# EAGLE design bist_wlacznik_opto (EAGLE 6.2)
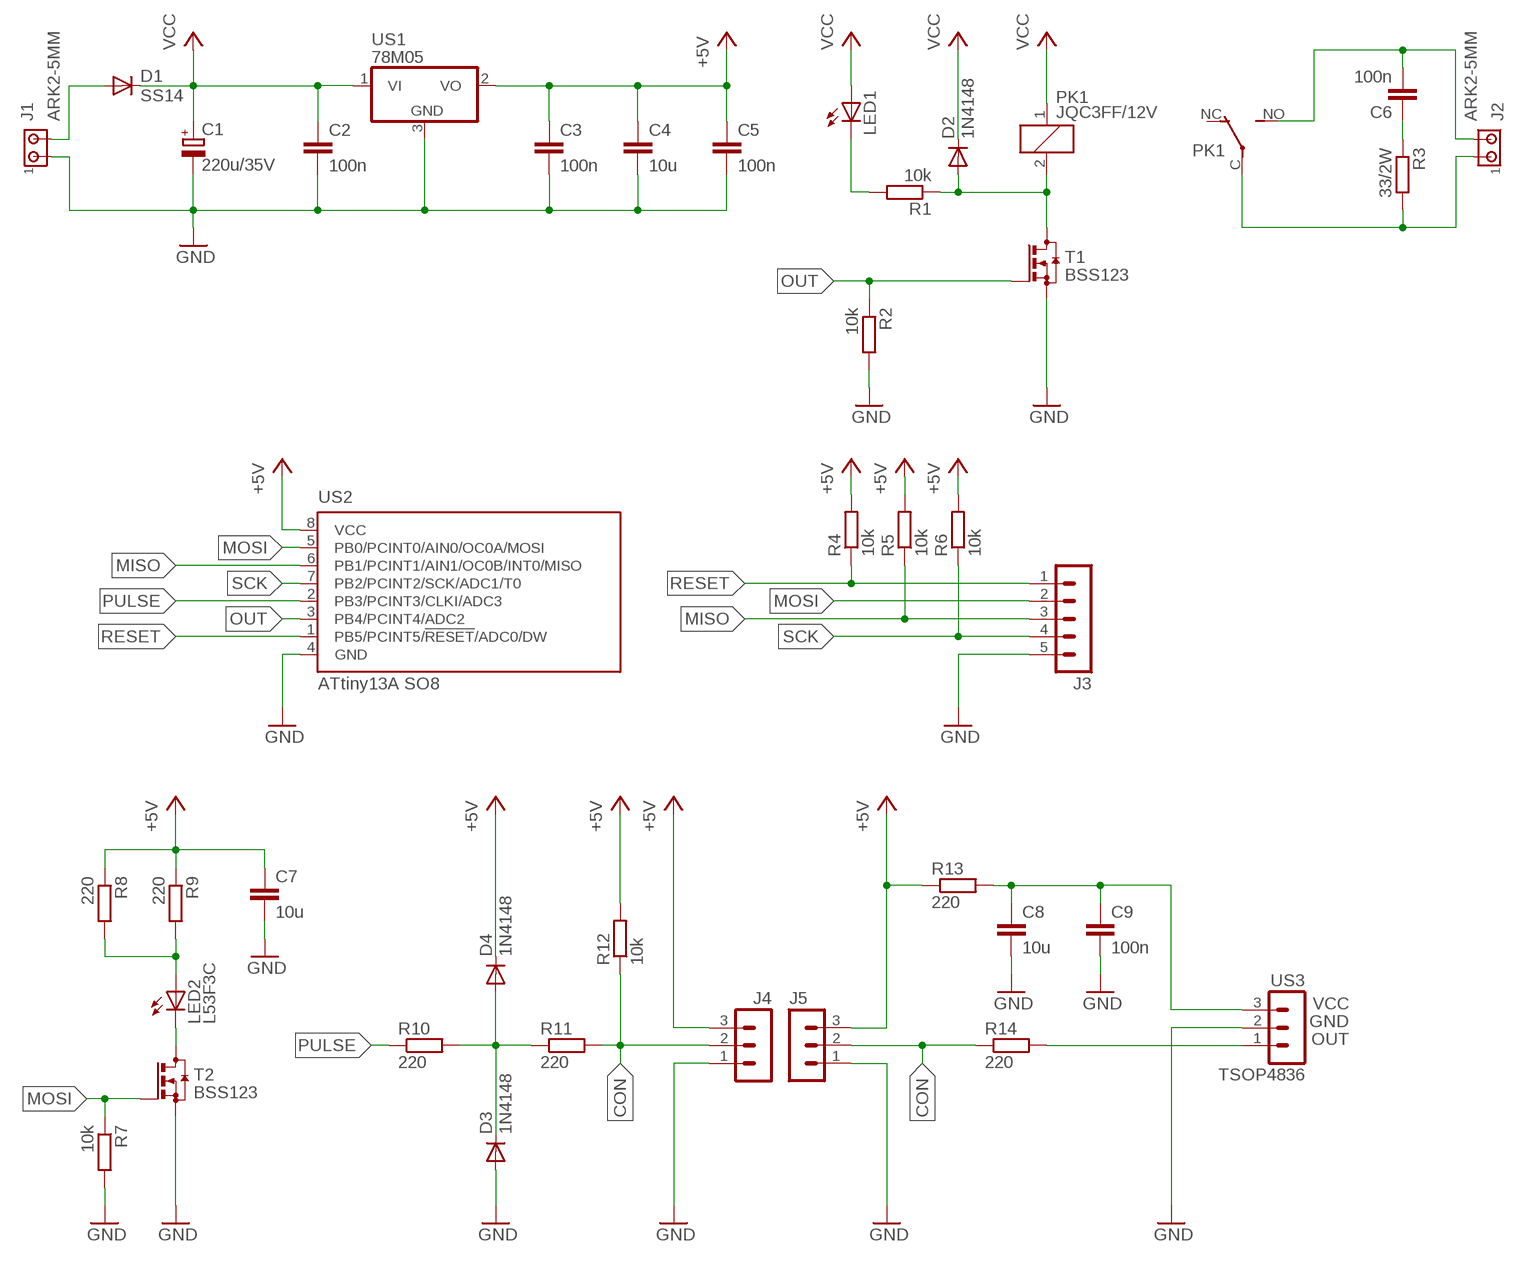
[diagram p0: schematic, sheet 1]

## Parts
C1  220u/35V  CPOL-EUE3.5-8  [E3,5-8]
C2  100n  C-EUC0805  [C0805]
C3  100n  C-EUC0805  [C0805]
C4  10u  C-EUC0805  [C0805]
C5  100n  C-EUC0805  [C0805]
C6  100n  C-EU102_152-062X184  [C102_152-062X184]
C7  10u  C-EUC0805  [C0805]
C8  10u  C-EUC0805  [C0805]
C9  100n  C-EUC0805  [C0805]
D1  SS14  DIODE-DO214AC  [DO214AC]
D2  1N4148  DIODE-MINIMELF  [MINIMELF]
D3  1N4148  DIODE-MINIMELF  [MINIMELF]
D4  1N4148  DIODE-MINIMELF  [MINIMELF]
J1  ARK2-5MM  [2PIN-5MM]
J2  ARK2-5MM  [2PIN-5MM]
J3  MA05-1  [MA05-1]
J4  MA03-1  [MA03-1]
J5  MA03-1  [MA03-1]
LED1  LEDCHIP-LED0805  [CHIP-LED0805]
LED2  L53F3C  LED5MM  [LED5MM]
PK1  JQC3FF/12V  PK_POJED-JQC-3FG  [PK_POJED_JQC-3FG]
R1  10k  R-EU_R0805  [R0805]
R2  10k  R-EU_M0805  [M0805]
R3  33/2W  R-EU_0617/5V  [0617V]
R4  10k  R-EU_R0805  [R0805]
R5  10k  R-EU_R0805  [R0805]
R6  10k  R-EU_R0805  [R0805]
R7  10k  R-EU_M0805  [M0805]
R8  220  R-EU_M0805  [M0805]
R9  220  R-EU_M0805  [M0805]
R10  220  R-EU_M0805  [M0805]
R11  220  R-EU_M0805  [M0805]
R12  10k  R-EU_R0805  [R0805]
R13  220  R-EU_M0805  [M0805]
R14  220  R-EU_M0805  [M0805]
T1  BSS123  [SOT23]
T2  BSS123  [SOT23]
US1  78M05  7806DT  [TO252]
US2  ATtiny13A SO8  TINY13V-10SSU  [8S1]
US3  TSOP4836  MA03-1  [MA03-1]

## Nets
+5V: C3.1 C4.1 C5.1 C7.1 D4.C J4.3 J5.3 R4.2 R5.2 R6.2 R8.1 R9.1 R12.2 R13.1 US1.2(VO) US2.8(VCC)
CON: J4.2 J5.2 R11.2 R12.1 R14.1
GND: C1.- C2.2 C3.2 C4.2 C5.2 C7.2 C8.2 C9.2 D3.A J1.P$1 J3.5 J4.1 J5.1 R2.2 R7.2 T1.2(S) T2.2(S) US1.3(GND) US2.4(GND) US3.2
MISO: J3.3 R5.1 US2.6(PB1/PCINT1/AIN1/OC0B/INT0/MISO)
MOSI: J3.2 R7.1 T2.1(G) US2.5(PB0/PCINT0/AIN0/OC0A/MOSI)
N$1: D1.A J1.P$2
N$2: LED1.C R1.2
N$4: LED2.K(C) T2.3(D)
N$5: LED2.A R8.2 R9.2
N$6: C8.1 C9.1 R13.2 US3.3
N$7: R14.2 US3.1
N$8: D3.C D4.A R10.2 R11.1
N$9: C6.1 R3.1
N$10: J2.P$1 PK1.C(COM) R3.2
N$11: C6.2 J2.P$2 PK1.NO
N$12: D2.A PK1.2 R1.1 T1.3(D)
OUT: R2.1 T1.1(G) US2.3(PB4/PCINT4/ADC2)
PULSE: R10.1 US2.2(PB3/PCINT3/CLKI/ADC3)
RESET: J3.1 R4.1 US2.1(PB5/PCINT5/!RESET!/ADC0/DW)
SCK: J3.4 R6.1 US2.7(PB2/PCINT2/SCK/ADC1/T0)
VCC: C1.+ C2.1 D1.C D2.C LED1.A PK1.1 US1.1(VI)
Unconnected: PK1.NC

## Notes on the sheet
- VCC
- GND
- OUT

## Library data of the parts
C1 = rcl:CPOL-EU: POLARIZED CAPACITOR, European symbol
C2-C5 C7-C9 = rcl:C-EU: CAPACITOR, European symbol
C6 = resistor:C-EU: CAPACITOR, European symbol
D1-D4 = diode:DIODE-: DIODE
J1 J2 = zlacza_futrzak:ARK2: ARK 2
J3 = zlacza_futrzak:MA05-1: PIN HEADER; OC_FARNELL: unknown; OC_NEWARK: unknown
J4 J5 = con-lstb:MA03-1: PIN HEADER; OC_FARNELL: unknown; OC_NEWARK: unknown
LED1 LED2 = led:LED: LED
PK1 = inne_futrzak:PK_POJED
R1 R2 R4-R14 = rcl:R-EU_: RESISTOR, European symbol
R3 = resistor:R-EU_: RESISTOR, European symbol
T1 T2 = transistor-small-signal:BSS123: N-CHANNEL MOS FET
US1 = linear:78*: Positive VOLTAGE REGULATOR Source: http://cache.national.com/ds/LM/LM78L05.pdf http://www.fairchildsemi.com/ds/LM/LM7805.pdf
US2 = atmel:TINY13: 8-bit AVR Microcontroller with 1K Bytes In-System Programmable Flash Source: http://www.atmel.com/dyn/resources/prod_documents/2535S.pdf; MPN: ATTINY13V-10SSU; OC_FARNELL: 1455135; OC_NEWARK: 58M3773
US3 = zlacza_futrzak:MA03-1: PIN HEADER; OC_FARNELL: unknown; OC_NEWARK: unknown

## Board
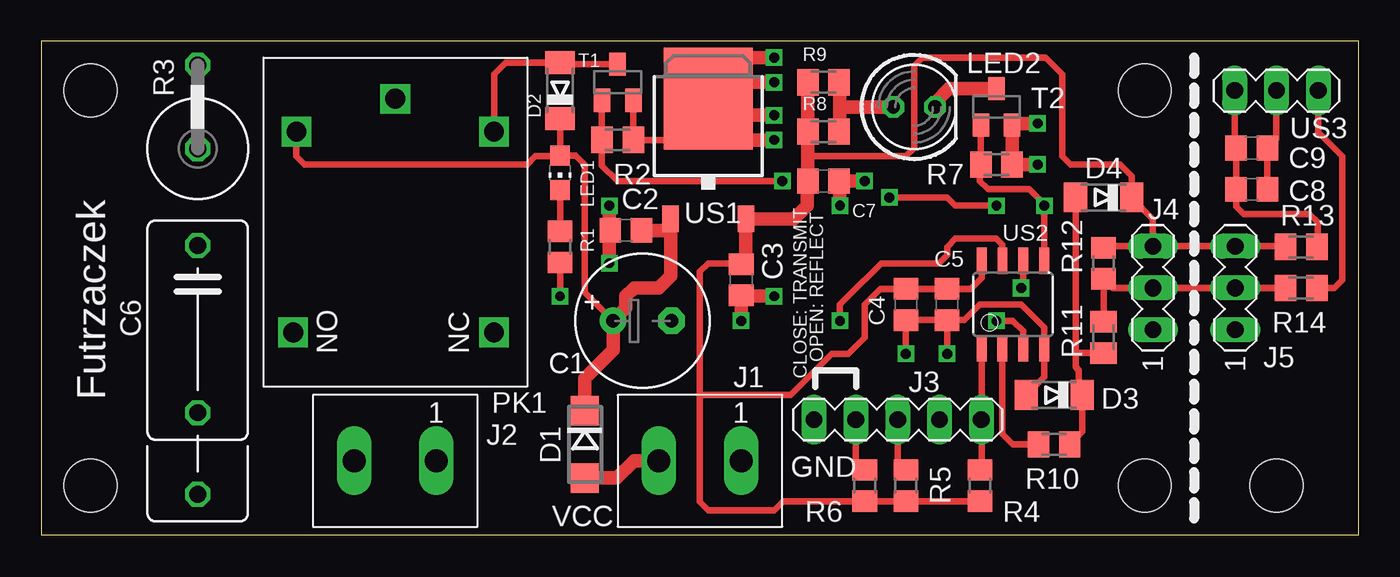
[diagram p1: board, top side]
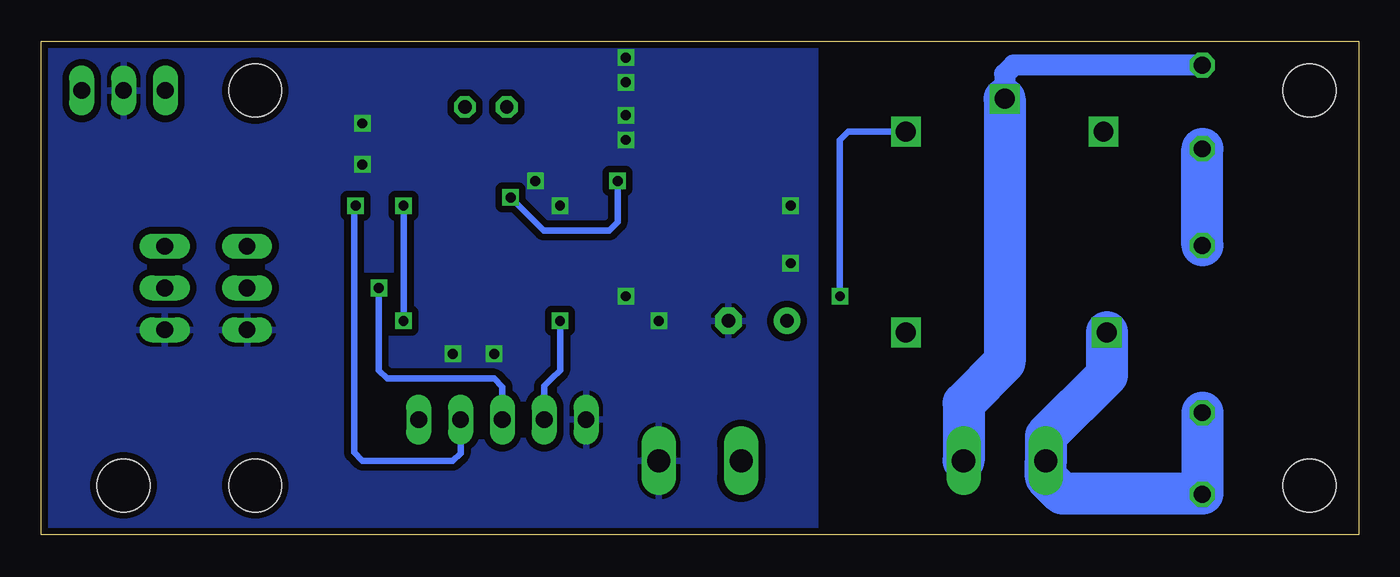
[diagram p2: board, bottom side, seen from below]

Size 80 x 30 mm. Coordinates in mm from the lower left corner, seen from the top.
Outline: 0,0 80,0 80,30 0,30 0,0
Copper layers (1*16): Top 0.035mm / dielectric 1.5mm / Bottom 0.035mm
Design rules: minimum track width 10mil, minimum drill 23mil, track to track 8mil, track to pad 8mil, pad to pad 8mil, via to via 8mil, smd to smd 8mil, copper to edge 10mil, drill to drill 8mil, minimum pad ring 10mil, minimum via ring 8mil, stop-mask expansion 4mil, vias tented up to drill 0mil, thermal gap 10mil
Holes 3.2 mm at 3,3 3,27 75,3 67,27 67,3

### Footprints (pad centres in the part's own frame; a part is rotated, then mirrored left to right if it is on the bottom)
E3,5-8 = drill 0.813 pad 1.6: + -1.778,0 | drill 0.813 pad 1.6 octagon: - 1.778,0
C0805 = smd 1.3 x 1.5: 1 -0.95,0; 2 0.95,0
C102_152-062X184 = drill 1.016 octagon: 1 -5.08,0; 2 5.08,0; 3 10.033,0
DO214AC = smd 1.8 x 1.7: A 2.05,0; C -2.05,0
MINIMELF = smd 1.4 x 1.8: A 1.7,0; C -1.7,0
2PIN-5MM = drill 1.4 long: P$1 -2.5,0; P$2 2.5,0
MA05-1 = drill 1.016 long: 1 -5.08,0; 2 -2.54,0; 3 0,0; 4 2.54,0; 5 5.08,0
MA03-1 = drill 1.016 long: 1 -2.54,0; 2 0,0; 3 2.54,0
CHIP-LED0805 = smd 1.2 x 1.2: A 0,-1.05; C 0,1.05
LED5MM = drill 0.813 octagon: A -1.27,0; K 1.27,0
PK_POJED_JQC-3FG = drill 1.2 square: 1 5.5,6; 2 5.5,-6; C 7.5,0; NC -6.7,-6; NO -6.7,6.2
R0805 = smd 1.3 x 1.5: 1 -0.95,0; 2 0.95,0
M0805 = smd 1.3 x 1.6: 1 -0.95,0; 2 0.95,0
0617V = drill 1.016 octagon: 1 -2.54,0; 2 2.54,0
SOT23 = smd 1 x 1.4: 1 -0.95,-1.1; 2 0.95,-1.1; 3 0,1.1
TO252 = smd 1 x 1.6: 1 -2.28,-4.8; 2 2.28,-4.8 | smd 5.4 x 6.2: 3 0,2.5
8S1 = smd 0.6 x 1.6: 1 -1.905,-2.654; 2 -0.645,-2.654; 3 0.625,-2.654; 4 1.895,-2.654; 5 1.905,2.654; 6 0.635,2.654; 7 -0.635,2.654; 8 -1.905,2.654

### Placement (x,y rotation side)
C1  36.5,13 0 top
C2  35.5,18.5 180 top
C3  42.5,15.5 270 top
C4  52.5,14 270 top
C5  55,14 270 top
C6  9.5,12.5 270 top
C7  47.5,21.5 0 top
C8  73.5,21 0 top
C9  73.5,23.5 0 top
D1  33,5.5 270 top
D2  31.5,27 90 top
D3  61.5,8.5 180 top
D4  64.5,20.5 180 top
J1  40,4.5 180 top
J2  21.5,4.5 180 top
J3  52,7 180 top
J4  67.5,15 90 top
J5  72.5,15 90 top
LED1  31.5,22 180 top
LED2  53,26 0 top
PK1  21.5,19 90 top
R1  31.5,17.5 90 top
R2  35,24 0 top
R3  9.5,26 90 top
R4  57,3 270 top
R5  52.5,3 270 top
R6  50,3 270 top
R7  58,22.5 0 top
R8  47.5,24.5 0 top
R9  47.5,27.5 0 top
R10  61.5,5.5 0 top
R11  64.5,12 90 top
R12  64.5,16.5 90 top
R13  76.5,17.5 0 top
R14  76.5,15 0 top
T1  35,27.5 0 top
T2  58,26 0 top
US1  40.5,24 0 top
US2  59,14 0 top
US3  75,27 180 top

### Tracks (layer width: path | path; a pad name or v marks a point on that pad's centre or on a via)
+5V
  Top 0.406: R13.1 75.51,17.54 J5.3 J4.3 | 40,8.5 40,2 40.5,1.5 44.5,1.5 45.05,2.05 R6.2 R5.2 R4.2 | 40,8.5 40,16 40.5,16.5 41.95,16.5 C3.1 | 40,8.5 45.5,8.5 47.96,10.96 48,11 49,11 50,12 50,14 50.95,14.95 C4.1 C5.1 56.45,14.95 57.09,15.6 US2.8 | J4.3 64.59,17.54 R12.2 | 46.55,23 52.5,23 53,23.5 53,28.5 53.5,29 61,29 62,28 62,23 62.5,22.5 65.5,22.5 66.2,21.8 D4.C 67.5,19.2 J4.3
  Top 0.813: R9.1 R8.1 46.55,23 C7.1 46.5,21.45 46.5,20 45.7,19.2 US1.2 42.78,16.73 C3.1
CON
  Top 0.406: R14.1 J5.2 J4.2 65.05,15 R12.1 R11.2
GND  (via drill 0.6)
  Top 0.406: T1.2 R2.2 40.5,24 | US3.2 75,24.05 C9.2 C8.2 | v52.5,11 C4.2 C5.2 | v55,11 C5.2 | D3.A 60.9,9.6 US2.4 60.9,12.61 59.5,14 57,14 56.05,13.05 C5.2
  Top 0.813: v44.5,24 40.5,24 40.5,25.5 | 40.5,25.5 US1.3 40.5,27.5 | v44.5,25.5 40.5,25.5 | v44.5,27.5 40.5,27.5 | v44.5,29 41,29 40.5,28.5 40.5,27.5 | v34.5,20 34.5,18.55 C2.2 34.5,18.45 v34.5,16.5 | 42.45,14.5 C3.2 | v42.5,13 C3.2 | v48.5,20 48.5,21.45 C7.2 v50,21.5 | v60.5,25 59.05,25 T2.2 R7.2 v60.5,22.5 | v44.5,14.5 42.55,14.5 C3.2
  pour Bottom (isolate 0.406): 80,0 80,30 33,30 33,0
MISO  (via drill 0.6)
  Top 0.406: US2.6 59.63,15.13 v59.5,15 | J3.3 52,4.45 R5.1
  Bottom 0.406: J3.3 52,9 52.5,9.5 59,9.5 59.5,10 v59.5,15
MOSI  (via drill 0.6)
  Top 0.406: T2.1 R7.1 57,22.45 57,21.5 57.5,21 60,21 60.91,20.09 v60.91,20 US2.5
  Bottom 0.406: J3.2 54.54,4.96 55,4.5 60.5,4.5 61,5 61,19.91 v60.91,20
N$1
  Top 0.813: D1.A 34.95,3.45 36,4.5 J1.P$2
N$2
  Top 0.406: R1.2 LED1.C
N$4
  Top 0.813: T2.3 55.1,27.1 54.27,26.27 LED2.K
N$5
  Top 0.813: LED2.A 48.5,26 | 48.5,26 48.5,24.55 R8.2 | 48.5,26 48.5,27.45 R9.2
N$6
  Top 0.406: US3.3 72.46,23.59 C9.1 C8.1 72.55,19.95 73,19.5 77,19.5 77.5,19 77.5,17.55 R13.2
N$7
  Top 0.406: R14.2 78.5,15 79,15.5 79,23 77.54,24.46 US3.1
N$8
  Top 0.406: R10.2 63.2,6.25 D3.C 63,8.7 63,10 62.8,10.2 62.8,11 | D4.A 62.8,11 | R11.1 62.85,11.05 62.8,11
N$9
  Bottom 2.54: C6.1 R3.1
N$10
  Bottom 1.27: R3.2 20.96,28.54 21.5,28 PK1.C
  Bottom 2.54: PK1.C 21.5,10.5 24,8 J2.P$1
N$11
  Bottom 2.54: PK1.NO 15.3,9.7 19,6 J2.P$2 19,3.5 18,2.5 9.5,2.5 C6.2
N$12  (via drill 0.6)
  Top 0.406: T1.3 31.6,28.6 D2.A 28.2,28.7 27.5,28 PK1.2 | v31.5,14.5 R1.1
  Bottom 0.406: PK1.2 31,24.5 31.5,24 v31.5,14.5
OUT  (via drill 0.6)
  Top 0.406: T1.1 R2.1 34.05,22.45 35,21.5 v45,21.5 | US2.3 59.62,12.38 59,13 v58,13 | v51.5,20.5 55,20.5 55.5,20 v58,20
  Bottom 0.406: v45,21.5 45,19 45.5,18.5 49.5,18.5 v51.5,20.5 | v58,20 v58,13
PULSE
  Top 0.406: US2.2 58.35,6.14 59,5.5 R10.1
RESET
  Top 0.406: US2.1 57.09,7.01 | 57.09,7.01 J3.1 | 57.09,7.01 57.09,4.04 R4.1
SCK  (via drill 0.6)
  Top 0.406: US2.7 58.37,17.64 58,18 55.5,18 55,17.5 55,17 54.5,16.5 51,16.5 49,14.5 48.5,14 v48.5,13 | R6.1 50.05,3.95 49.5,4.5 49.46,4.54 J3.4
  Bottom 0.406: v48.5,13 48.5,10 49,9.5 49.46,9.04 J3.4
VCC
  Top 0.406: PK1.1 15.5,23 16,22.5 29.5,22.5 30,23 31.45,23 LED1.A | LED1.A D2.C | LED1.A 32.45,23.05 33,22.5 33,14.72 C1.+
  Top 0.813: D1.C 33,9.5 34.72,11.22 C1.+ 35.5,13.78 35.5,14.5 36,15 37.5,15 38.22,15.72 38.22,18.5 | US1.1 38.22,18.5 | C2.1 38.22,18.5

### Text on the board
tPlace: CLOSE: TRANSMIT | OPEN: REFLECT | Futrzaczek | GND | VCC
